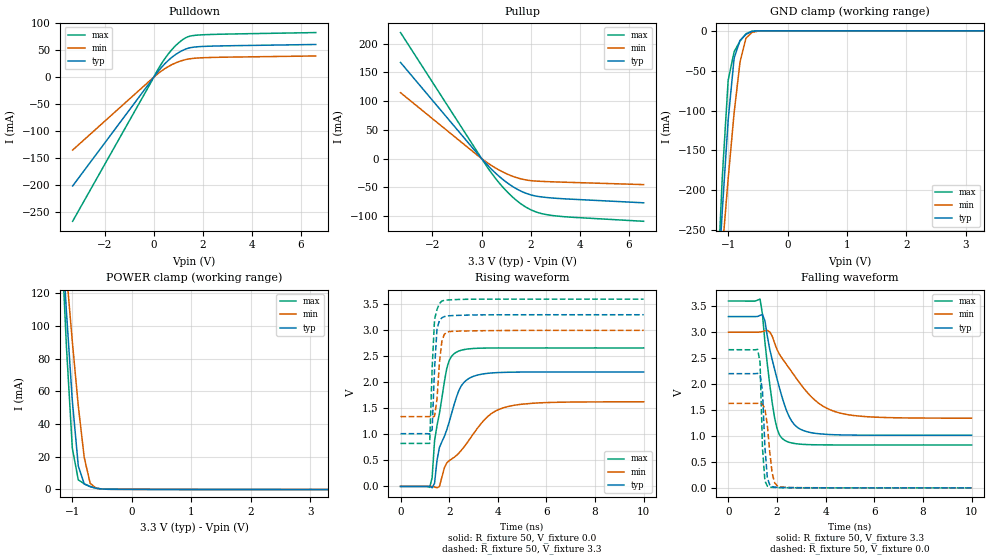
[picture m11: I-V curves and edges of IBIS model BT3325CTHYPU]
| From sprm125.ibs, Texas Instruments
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[Model]   BT3325CTHYPU
Model_type   I/O
Vinh = 2.00
Vinl = 0.80
Enable   Active-Low
Polarity   Non-Inverting
| signals   A, GZ, Y
Vmeas = 1.5
|   typ   min   max
C_comp   1.5797p   1.5046p   1.7659p
|   typ   min   max
[Temperature Range]   25   -40   125
|   typ   min   max
[Voltage Range]   3.30V   3.00V   3.60V
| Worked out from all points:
|   slope of the pulldown table from 0 to 0.495 V, typ, clamps not added: 18.4 ohm
|   slope of the pullup table from 0 to 0.495 V, typ, clamps not added: 22.1 ohm
|   GND clamp passes 1 mA (typ) near -0.60 V on its own axis
|   POWER clamp passes 1 mA (typ) near -0.63 V on its own axis
|   rising waveform, R_fixture 50, V_fixture 0.0: 20-80 % time 848ps typ, 1.71ns min, 497ps max; typ from 0 V to 2.2 V
|   falling waveform, R_fixture 50, V_fixture 3.3: 20-80 % time 774ps typ, 1.6ns min, 432ps max; typ from 3.3 V to 1.01 V
|   rising waveform, R_fixture 50, V_fixture 3.3: 20-80 % time 143ps typ, 171ps min, 144ps max; typ from 1.01 V to 3.3 V
|   falling waveform, R_fixture 50, V_fixture 0.0: 20-80 % time 148ps typ, 218ps min, 120ps max; typ from 2.2 V to 0 V
[Pulldown]
|   Voltage   I(typ)   I(min)   I(max)
-3.3V     -201.5mA   -134.9mA   -267mA
200mV     11.94mA    7.607mA    16.41mA
600mV     31.43mA    19.94mA    43.44mA
800mV     39.06mA    24.71mA    54.18mA
1.1V      47.98mA    30.18mA    66.99mA
1.4V      53.8mA     33.69mA    75.19mA
1.9V      56.89mA    36.01mA    78.53mA
6.6V      60.8mA     39.52mA    82.88mA
[GND_clamp]
|   Voltage   I(typ)   I(min)   I(max)
-3.3V     -3.359A    -2.535A    -4.36A
-1.2V     -355mA     -371.1mA   -350mA
-1.1V     -226.8mA   -276.2mA   -185.1mA
-1V       -111.9mA   -185.5mA   -62.01mA
-900mV    -34.22mA   -103mA     -26.29mA
-800mV    -12.03mA   -38.74mA   -12.65mA
-700mV    -4.384mA   -9.072mA   -3.684mA
-600mV    -848.8uA   -2.124mA   -417.4uA
-400mV    -4.328uA   -46.41uA   -434.3nA
3.3V      222pA      2.083uA    133.2pA
[Pullup]
|   Voltage   I(typ)   I(min)   I(max)
-3.3V     167.1mA    114.5mA    219.1mA
-200mV    10mA       6.709mA    13.35mA
300mV     -14.08mA   -9.224mA   -19.1mA
600mV     -26.64mA   -17.31mA   -36.28mA
900mV     -37.6mA    -24.2mA    -51.46mA
1.2V      -46.92mA   -29.85mA   -64.58mA
1.5V      -54.52mA   -34.2mA    -75.6mA
1.8V      -60.33mA   -37.21mA   -84.43mA
2.1V      -64.3mA    -38.86mA   -91.01mA
2.7V      -68.04mA   -40.24mA   -98mA
3.6V      -70.63mA   -41.51mA   -101.9mA
6.6V      -77.05mA   -45.41mA   -109.2mA
[POWER_clamp]
|   Voltage   I(typ)   I(min)   I(max)
-3.3V     1.576A     1.191A     2.045A
-1.2V     169.8mA    177.9mA    166.5mA
-1.1V     109.3mA    133.2mA    87.92mA
-1V       54.23mA    90.45mA    25.1mA
-900mV    14.35mA    51.17mA    5.826mA
-800mV    3.269mA    19.53mA    3.421mA
-700mV    1.617mA    3.736mA    1.806mA
-600mV    705uA      738uA      676uA
-500mV    198.5uA    185uA      148.6uA
3.3V      -108.3uA   -67.78uA   -162.1uA
[Ramp]
|   I(typ)   I(min)   I(max)
dV/dt_r   1.320/0.846n   0.976/1.712n   1.597/0.499n
dV/dt_f   1.372/0.778n   0.995/1.602n   1.664/0.434n
[Rising Waveform]
R_fixture = 50
V_fixture = 0.0
|  pu_on
|  TIME   V(typ)   V(min)   V(max)
0s        2nV        12nV       1nV
1.2ns     2.163mV    1.088mV    -18.76mV
1.3ns     -25.5mV    1.603mV    168.2mV
1.4ns     61.18mV    -9.166mV   879.3mV
1.6ns     747.7mV    -1.531mV   1.404V
1.9ns     1.085V     450mV      2.265V
2.3ns     1.717V     595.5mV    2.581V
2.9ns     2.097V     946.6mV    2.648V
4.3ns     2.193V     1.521V     2.662V
10ns      2.2V       1.626V     2.662V
[Falling Waveform]
R_fixture = 50
V_fixture = 3.3
V_fixture_min = 3.0
V_fixture_max = 3.6
|  pd_on
|  TIME   V(typ)   V(min)   V(max)
0s        3.3V       3V         3.6V
1.3ns     3.323V     3.002V     3.636V
1.4ns     3.339V     3.011V     3.341V
1.5ns     3.218V     3.025V     2.81V
1.9ns     2.281V     2.788V     1.345V
2.1ns     1.922V     2.573V     1.019V
2.3ns     1.607V     2.434V     919.1mV
2.9ns     1.145V     2.04V      844.4mV
4.4ns     1.023V     1.466V     826.9mV
10ns      1.014V     1.342V     826.4mV
[Rising Waveform]
R_fixture = 50
V_fixture = 3.3
V_fixture_min = 3.0
V_fixture_max = 3.6
|  pd_off
|  TIME   V(typ)   V(min)   V(max)
0s        1.014V     1.342V     826.4mV
1.2ns     1.007V     1.343V     827.5mV
1.3ns     1.093V     1.327V     2.263V
1.4ns     2.27V      1.349V     3.214V
1.5ns     3.031V     1.673V     3.401V
1.6ns     3.188V     2.376V     3.515V
1.7ns     3.242V     2.79V      3.564V
1.8ns     3.264V     2.922V     3.577V
2.1ns     3.283V     2.98V      3.588V
10ns      3.3V       3V         3.6V
[Falling Waveform]
R_fixture = 50
V_fixture = 0.0
|  pu_off
|  TIME   V(typ)   V(min)   V(max)
0s        2.2V       1.626V     2.662V
1.2ns     2.206V     1.629V     2.668V
1.3ns     2.178V     1.635V     2.417V
1.4ns     1.865V     1.612V     768.6mV
1.5ns     784.7mV    1.521V     134.6mV
1.6ns     191.8mV    1.208V     33.88mV
1.8ns     25.86mV    278.8mV    9.419mV
1.9ns     14.36mV    98.04mV    7.25mV
2.1ns     7.451mV    23.25mV    4.834mV
10ns      518nV      6.451uV    530nV
